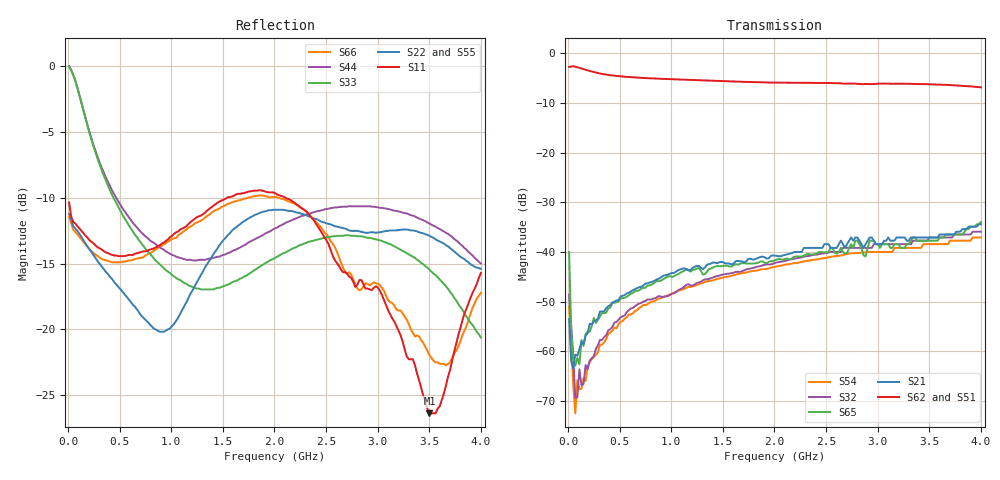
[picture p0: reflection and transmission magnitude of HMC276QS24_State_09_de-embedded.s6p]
! Hittite Microwave Corporation
! 20 Alpha Road
! Chelmsford, MA 01824
! Tel: 978-250-3343
! Fax: 978-250-3373
! Device: HMC276QS24, 0.7-3.0 GHz, GaAS MMIC 4x2 Switch Matrix in 24-lead QSOP package
! Misc: Data was de-embedded to package pins.
!  Port 1 = OP1
!  Port 2 = VL
!  Port 3 = VH
!  Port 4 = HH
!  Port 5 = HL
!  Port 6 = OP2
!  Vdd = +5 V
!  Vctl = 0 V[Logic 0] / +5 V[Logic 1]
!  State 09,  HL to OP1,  VL to OP2
!  Control Lines (Logic)
!  HV 1 = 1, Tone 1 = 0
!  HV 2 = 0, Tone 2 = 0
!  Data reformated to new Touchstone file format - Wed Jan 10 15:20:20 2007
# MHz S DB R 50
! 6 Port Network Data
! freq  dbS11  angS11  dbS12  angS12  dbS13  angS13  dbS14  angS14
!  dbS15  angS15  dbS16  angS16
!  dbS21  angS21  dbS22  angS22
!  dbS23  angS23  dbS24  angS24  dbS25  angS25  dbS26  angS26
!  dbS31  angS31  dbS32  angS32  dbS33  angS33  dbS34  angS34
!  dbS35  angS35  dbS36  angS36
!  dbS41  angS41  dbS42  angS42
!  dbS43  angS43  dbS44  angS44  dbS45  angS45  dbS46  angS46
!  dbS51  angS51  dbS52  angS52  dbS53  angS53  dbS54  angS54
!  dbS55  angS55  dbS56  angS56
!  dbS61  angS61  dbS62  angS62
!  dbS63  angS63  dbS64  angS64  dbS65  angS65  dbS66  angS66
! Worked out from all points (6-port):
!   201 points, 10 MHz to 4 GHz, reference 50 ohm
!   strongest paths, dB at 10 MHz, 1.008 GHz, 2.005 GHz, 3.002 GHz, 4 GHz:
!     S62: -2.7, -5.2, -5.9, -6.1, -6.8
!     S51: -2.8, -5.3, -6.0, -6.2, -6.9
!     S21: -53.5, -44.2, -40.7, -38.4, -34.4
!     S65: -40.0, -45.0, -41.6, -38.4, -34.0
!     S32: -48.6, -48.4, -42.2, -38.4, -35.9
!     S54: -51.1, -48.4, -43.0, -40.0, -37.1
!   lowest |S11| = -26.4 dB at 3.501 GHz (marker M1), VSWR 1.10, Z = 50.3 + j4.81 ohm
!   |S11| at or under -10 dB: start of sweep to 1.537 GHz; 2.11 GHz to end of sweep
